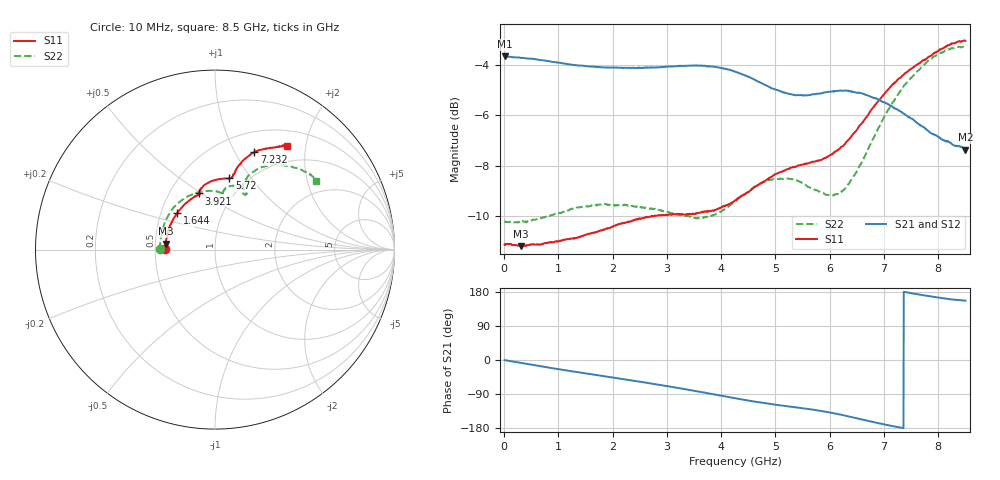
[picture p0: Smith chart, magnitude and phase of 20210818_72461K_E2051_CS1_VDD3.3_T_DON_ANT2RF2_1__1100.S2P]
!Agilent Technologies,E5071C,MY46417908,A.11.23
!Date: Wed Aug 18 14:26:28 2021
!Data & Calibration Information:
!Freq	S11:SOLT2(ON)	S21:SOLT2(ON)	S12:SOLT2(ON)	S22:SOLT2(ON)
!PortZ  Port1:50+j0  Port2:50+j0
!Above PortZ is port z conversion or system Z0 setting when saving the data.
!When reading, reference impedance value at option line is always used.
# Hz S dB R 50
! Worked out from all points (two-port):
!   1601 points, 10 MHz to 8.5 GHz, reference 50 ohm
!   highest |S21| = -3.66 dB at 10 MHz (marker M1); lowest = -7.4 dB at 8.5 GHz (marker M2)
!   |S21| within 3 dB of the highest: start of sweep to 7.829 GHz
!   lowest |S11| = -11.2 dB at 312.5 MHz (marker M3), VSWR 1.76, Z = 28.5 + j1.99 ohm
!   |S11| at or under -10 dB: start of sweep to 2.767 GHz; 2.784389 GHz to 2.794564 GHz (10.17 MHz wide, 0.365 % of centre)
!   |S22| runs from -10.3 to -3.3 dB; largest |S21 - S12| = 0.0021
!   S11 on the Smith chart (normalised r, x): 10 MHz: 0.57, +0.00; 1.644 GHz: 0.61, +0.27; 3.921 GHz: 0.70, +0.49; 5.72 GHz: 0.83, +0.79; 7.232 GHz: 0.73, +1.20; 8.5 GHz: 0.73, +1.67
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1e7  -11.14 179.6  -3.66 -0.4  -3.65 -0.4  -10.21 179.7
3.124562e8  -11.20 173.3  -3.73 -7.8  -3.72 -7.8  -10.23 170.2
9.332875e8  -11.04 158.1  -3.89 -22.6  -3.89 -22.6  -9.92 149.9
1.426769e9  -10.81 143.1  -4.03 -33.7  -4.03 -33.6  -9.64 132.2
1.644325e9  -10.68 136.3  -4.07 -38.4  -4.07 -38.4  -9.60 124.2
2.206788e9  -10.28 120.8  -4.12 -50.8  -4.12 -50.7  -9.56 105.3
2.843538e9  -9.98 109.6  -4.09 -65.2  -4.09 -65.2  -9.76 89.2
3.443144e9  -9.92 106.1  -4.03 -79.6  -4.02 -79.6  -10.04 82.8
3.920706e9  -9.75 105.9  -4.09 -92.0  -4.09 -92.0  -9.91 82.1
4.255e9  -9.39 104.3  -4.27 -100.8  -4.26 -100.9  -9.43 81.0
4.928894e9  -8.45 94.3  -4.93 -116.5  -4.93 -116.5  -8.56 72.0
5.671769e9  -7.86 79.3  -5.18 -130.6  -5.19 -130.6  -8.91 60.6
5.719525e9  -7.85 78.6  -5.17 -131.7  -5.18 -131.7  -8.96 60.3
6.032594e9  -7.57 76.4  -5.06 -139.4  -5.08 -139.5  -9.20 61.8
6.281988e9  -7.14 75.6  -5.02 -146.8  -5.02 -146.9  -8.92 64.4
6.658731e9  -6.12 73.7  -5.19 -159.1  -5.19 -159.1  -7.57 66.4
7.088538e9  -4.94 69.5  -5.58 -172.5  -5.59 -172.6  -5.76 61.6
7.231806e9  -4.65 68.0  -5.77 -176.4  -5.78 -176.5  -5.28 58.5
7.491812e9  -4.17 64.6  -6.12 176.7  -6.12 176.6  -4.54 53.0
7.937538e9  -3.51 59.1  -6.78 166.1  -6.77 166.0  -3.65 42.4
8.218769e9  -3.19 56.8  -7.09 160.4  -7.06 160.5  -3.37 37.2
8.5e9  -3.05 55.0  -7.37 156.6  -7.34 156.4  -3.33 34.0
